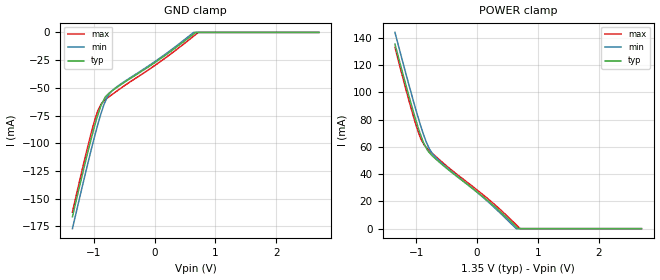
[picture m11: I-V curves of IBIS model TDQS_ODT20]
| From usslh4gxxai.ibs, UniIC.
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| MODEL TDQS_ODT20 (TDQS Terminator Model with 20ohm ODT, 800-2133Mbps)
[Model]   TDQS_ODT20
Model_type   Terminator
|   typ   min   max
|C_comp   1.035pF   0.986pF   1.103pF
C_comp_power_clamp   0.5175pF   0.4930pF   0.5515pF
C_comp_gnd_clamp   0.5175pF   0.4930pF   0.5515pF
| Note: C_comp changes when the ODT circuit is enabled.
[Voltage Range]   1.3500V   1.2830V   1.4250V
[Temperature Range]   45.0   95.0   -40.0
[GND Clamp]
|   Voltage   I(typ)   I(min)   I(max)
-1.35V    -166.3mA   -177.1mA   -162.2mA
-1.11V    -110.8mA   -121mA     -105.5mA
-990mV    -85.35mA   -94.61mA   -80.22mA
-935mV    -74.97mA   -83.31mA   -70.92mA
-885mV    -66.4mA    -73.78mA   -65.36mA
-810mV    -58.2mA    -62.2mA    -60.6mA
-785mV    -56.84mA   -58.97mA   -59.54mA
-680mV    -51.97mA   -51.62mA   -55.27mA
110mV     -23.21mA   -22.26mA   -25.7mA
640mV     -1.463mA   0A         -3.434mA
718mV     0A         0A         0A
2.7V      0A         0A         0A
[POWER Clamp]
|   Voltage   I(typ)   I(min)   I(max)
-1.35V    135.5mA    144.1mA    133.2mA
-1.11V    95.68mA    103.8mA    92.36mA
-990mV    77.3mA     84.75mA    74mA
-930mV    69.11mA    75.86mA    66.49mA
-885mV    63.46mA    69.61mA    62.66mA
-780mV    55.58mA    58.21mA    57.08mA
-730mV    53.18mA    54.8mA     55.01mA
-590mV    47.64mA    48.4mA     49.42mA
115mV     22.74mA    22.32mA    24.22mA
640mV     1.535mA    94.48uA    2.93mA
707mV     0A         0A         0A
2.7V      0A         0A         0A
